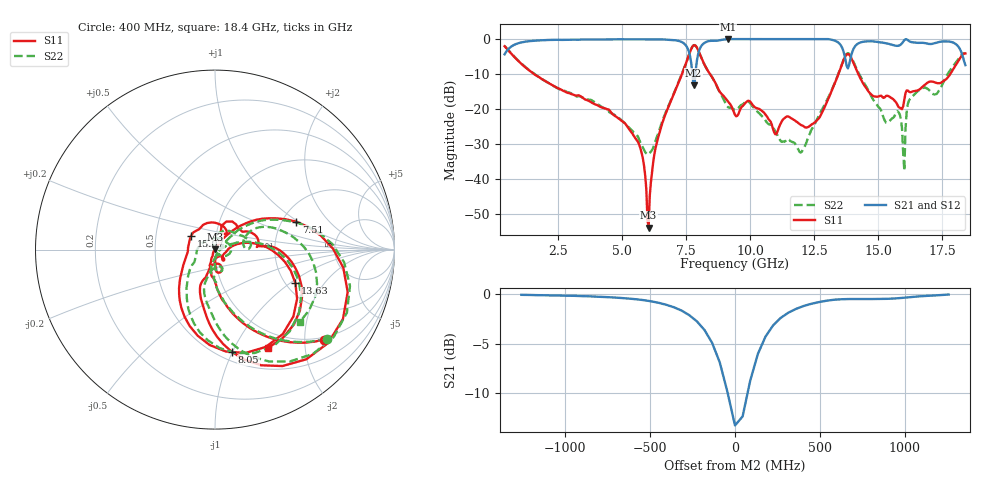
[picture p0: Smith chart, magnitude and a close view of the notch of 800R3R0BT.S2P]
!  American Technical Ceramics  Date:  10/25/10
!  One Norden Lane
!  Huntington Station,  NY.  11746-2102
!  Tel:  (631) 622-4700  Fax:  (631) 622-4748
!  Part Number  800R3R0BT.TXT  Mounting Orientation: Horizontal
!  Description: Ultra Low ESR Microwave Capacitor
!  Application: Coupling, Bypass, Tuning, DC Block, Filters, Matching
# GHZ S DB R 50
! Freq  |S11|  S11 Ph  |S21|  S21 Ph  |S12|  S12 Ph  |S22|  S22 Ph
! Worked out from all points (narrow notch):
!   401 points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, 400 MHz to 18.4 GHz, reference 50 ohm
!   highest |S21| = -0.01 dB at 9.13 GHz (marker M1); lowest = -13.2 dB at 7.78 GHz (marker M2)
!   notch at M2: 13.0 dB deep, 216 MHz wide at half that depth
!   lowest |S11| = -54.0 dB at 6.025 GHz (marker M3), VSWR 1.00, Z = 50.1 + j0.184 ohm
!   |S11| at or under -10 dB: 1.545 GHz to 7.33 GHz (5.785 GHz wide, 130 % of centre); 8.422 GHz to 13.44 GHz (5.02 GHz wide, 45.9 % of centre); 14.22 GHz to 17.81 GHz (3.594 GHz wide, 22.4 % of centre)
!   |S22| runs from -37.7 to -1.7 dB; largest |S21 - S12| = 0.0057
!   S11 on the Smith chart (normalised r, x): 400 MHz: 0.94, -2.48; 7.51 GHz: 2.38, +0.96; 8.05 GHz: 0.58, -1.00; 13.63 GHz: 2.25, -1.10; 15.07 GHz: 0.76, +0.12; 18.4 GHz: 0.77, -1.37
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0.4  -2.06 -39.4  -4.37 50.6  -4.39 50.6  -1.98 -38.5
1.3  -8.63 -74.5  -0.66 16.0  -0.68 16.1  -8.54 -73.2
3.415  -16.59 -97.3  -0.14 -6.8  -0.15 -6.8  -16.67 -94.3
5.53  -28.61 -110.3  -0.10 -21.1  -0.11 -21.0  -27.22 -85.0
6.025  -54.00 66.9  -0.07 -25.1  -0.06 -24.9  -32.95 -28.1
6.43  -27.36 57.0  -0.09 -28.7  -0.09 -28.6  -26.37 29.7
7.51  -6.40 19.0  -2.13 -56.3  -2.11 -56.2  -6.49 18.8
7.78  -1.82 -28.5  -13.21 -41.3  -13.20 -41.2  -1.78 -25.6
8.05  -4.76 -80.6  -2.40 2.3  -2.39 2.4  -4.77 -75.9
9.13  -17.87 -106.7  -0.01 -24.0  -0.01 -23.9  -19.53 -92.6
9.4  -21.71 -95.9  -0.01 -26.2  -0.01 -26.1  -20.26 -77.7
11.965  -24.55 -46.6  -0.01 -50.3  -0.01 -50.2  -32.48 -26.8
12.415  -24.34 -15.9  -0.01 -54.0  -0.01 -54.1  -25.59 14.1
13.63  -6.27 -22.7  -3.35 -83.0  -3.33 -83.1  -6.08 -20.3
14.125  -8.50 -119.8  -1.77 -37.6  -1.75 -37.7  -8.13 -110.3
15.07  -16.25 150.6  -0.94 -57.6  -0.92 -57.6  -19.91 -177.6
15.43  -16.47 90.7  -1.43 -59.7  -1.42 -59.9  -23.51 71.5
15.79  -19.47 56.3  -1.90 -54.3  -1.87 -54.4  -20.94 -5.6
15.97  -19.21 72.3  -0.75 -50.6  -0.73 -50.9  -32.66 -61.2
16.285  -15.16 41.8  -0.86 -62.1  -0.84 -62.2  -16.79 38.9
17.905  -8.86 -0.6  -0.96 -75.4  -0.94 -75.6  -7.90 13.8
18.4  -4.11 -61.8  -7.47 -71.3  -7.44 -71.3  -4.13 -40.7
